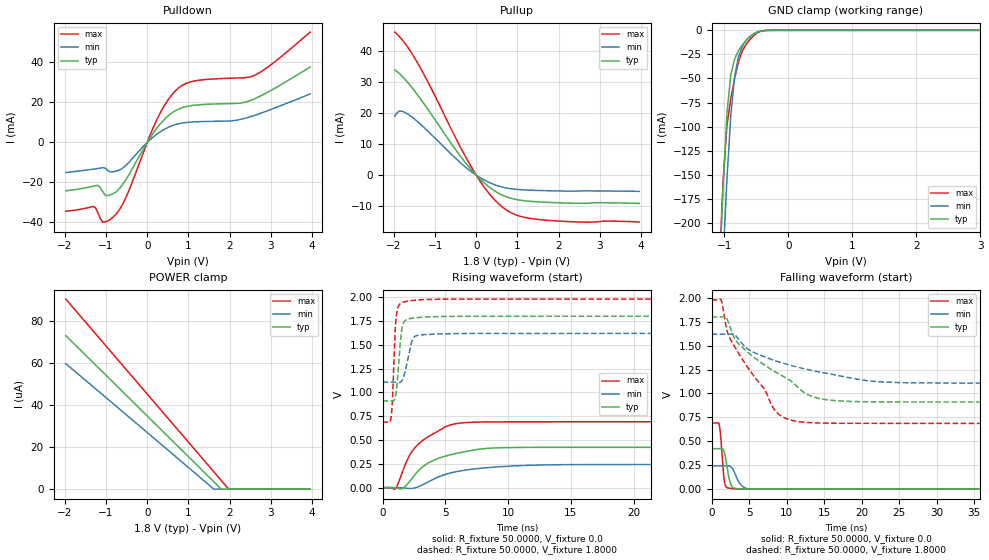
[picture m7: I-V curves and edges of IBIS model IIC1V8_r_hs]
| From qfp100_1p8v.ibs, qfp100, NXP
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[Model] IIC1V8_r_hs
|   Model IIC1V8_r_hs
| This model was characterised for following simulation conditions:
| External (pad) voltage:
|   - Typ: 1.8V,   - Min: 1.62V,   - Max: 1.98V
| Library cells for typ/min/max conditions are connected as defined below:
|  IO - External Pad
|  A - Core Input
|  EN - Output Buffer Enable
|  BOOST - vdde
|  EGP - vdd
|  EHS - vdd
|  ENZI - vdd
|  EPD - vdd
|  EPUN - gnd
|  ZI - NC
|  ZIF - NC
|  gnd - gnd
|  gnde - gnde
|  vdd - vdd
|  vdde - vdde
| All other pins connected to ground
Model_type I/O
Polarity   Non-Inverting
Enable   Active-Low
Vinl =   0.5400V
Vinh =   1.2600V
Vmeas =  0.9000V
Cref =   0.0F
Rref =   1.0000k
Vref =   0.0V
C_comp   3.6136pF   3.4665pF   3.7543pF
|C_comp_pullup   0.9376pF   0.9158pF   0.9440pF
|C_comp_pulldown   2.3253pF   2.4782pF   2.1796pF
[Model Spec]
| variable   typ   min   max
Vinh   0.5400V   0.4860V   0.5940V
Vinl   1.2600V   1.1340V   1.3860V
Vmeas   0.9000V   0.8100V   0.9900V
[Temperature Range]   25.0000   0.1250k   -40.0000
[Voltage Range]   1.8000V   1.6200V   1.9800V
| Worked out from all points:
|   slope of the pulldown table from 0 to 0.27 V, typ, clamps not added: 33.4 ohm
|   slope of the pullup table from 0 to 0.27 V, typ, clamps not added: 80.7 ohm
|   GND clamp passes 1 mA (typ) near -0.44 V on its own axis
|   rising waveform, R_fixture 50.0000, V_fixture 0.0: 20-80 % time 2.94ns typ, 3.7ns min, 2.37ns max; typ from 0 V to 0.423 V
|   rising waveform, R_fixture 50.0000, V_fixture 1.8000: 20-80 % time 334ps typ, 515ps min, 244ps max; typ from 0.91 V to 1.8 V
|   falling waveform, R_fixture 50.0000, V_fixture 0.0: 20-80 % time 581ps typ, 938ps min, 399ps max; typ from 0.423 V to 0 V
|   falling waveform, R_fixture 50.0000, V_fixture 1.8000: 20-80 % time 8.41ns typ, 11.2ns min, 5.74ns max; typ from 1.8 V to 0.91 V
[Pulldown]
|Voltage   I(typ)   I(min)   I(max)
-1.98V    -24.22mA   -15.04mA   -34.42mA
-1.32V    -21.94mA   -13.41mA   -32.06mA
-1.2V     -21.45mA   -13.05mA   -35.06mA
-1.08V    -24.63mA   -12.6mA    -39.9mA
-900mV    -26.23mA   -14.78mA   -38.53mA
-720mV    -24.07mA   -14.13mA   -34.99mA
-540mV    -19.33mA   -11.9mA    -28.53mA
300mV     8.856mA    5.096mA    14.12mA
720mV     16.26mA    9.117mA    26.48mA
1.14V     18.6mA     10.26mA    30.69mA
2.58V     21.55mA    13.34mA    33.32mA
3.96V     37.7mA     24.26mA    55.17mA
[Pullup]
|Voltage   I(typ)   I(min)   I(max)
-1.98V    33.82mA    18.95mA    45.98mA
-1.86V    32.54mA    20.66mA    44.41mA
-1.62V    29.1mA     19.25mA    40.23mA
-1.2V     21.63mA    14.45mA    30.58mA
-420mV    6.731mA    4.413mA    9.887mA
0V        -16.46nA   -7.885nA   -32.77nA
360mV     -4.265mA   -2.608mA   -6.666mA
660mV     -6.57mA    -3.917mA   -10.5mA
1.02V     -7.945mA   -4.606mA   -13.01mA
1.56V     -8.618mA   -4.934mA   -14.29mA
2.64V     -9.058mA   -5.064mA   -15.11mA
3.96V     -9.081mA   -5.209mA   -15.04mA
[GND_clamp]
|Voltage   I(typ)   I(min)   I(max)
-1.98V    -2.104A    -2.075A    -2.136A
-1.08V    -259.3mA   -333mA     -246.9mA
-1.02V    -161.8mA   -238.7mA   -157.1mA
-960mV    -86.75mA   -154.7mA   -99.47mA
-900mV    -45.96mA   -88.82mA   -71.06mA
-840mV    -29.91mA   -48mA      -50.26mA
-780mV    -21.16mA   -27.65mA   -32.99mA
-720mV    -15.17mA   -16.88mA   -21.27mA
-660mV    -10.57mA   -10.24mA   -14.57mA
-540mV    -3.796mA   -3.405mA   -5.301mA
-300mV    -21.69uA   -40.85uA   -23.15uA
3.96V     0A         0A         0A
[POWER_clamp]
|Voltage   I(typ)   I(min)   I(max)
-1.98V    73.06uA    59.72uA    90.42uA
1.62V     3.484uA    0A         8.225uA
1.8V      0A         0A         4.113uA
1.98V     0A         0A         0A
3.96V     0A         0A         0A
[Ramp]
| variable   typ   min   max
dV/dt_r  0.2537/2.9385n   0.1456/3.7026n   0.4146/2.3719n
dV/dt_f  0.5332/8.4056n   0.3066/11.2315n   0.7749/5.7392n
R_load = 50.0000
[Rising Waveform]
R_fixture= 50.0000
V_fixture= 0.0
V_fixture_min= 0.0
V_fixture_max= 0.0
|time   V(typ)   V(min)   V(max)
0s        583.8pV    50.78nV    39.11pV
1.054ns   -4.544mV   243uV      -9.405mV
1.612ns   -8.369mV   -2.334mV   175mV
2.288ns   86.03mV    -8.936mV   367.6mV
2.979ns   193.4mV    16.44mV    471mV
3.665ns   259.9mV    61.19mV    536.3mV
5.554ns   349.4mV    158.1mV    662.5mV
8.944ns   416.4mV    215.7mV    689.9mV
23.83ns   422.8mV    242.5mV    690.9mV
1us       422.9mV    242.6mV    691mV
[Rising Waveform]
R_fixture= 50.0000
V_fixture= 1.8000
V_fixture_min= 1.6200
V_fixture_max= 1.9800
|time   V(typ)   V(min)   V(max)
0s        910.3mV    1.108V     687.5mV
692.7ps   908.2mV    1.108V     745.4mV
790.9ps   905.2mV    1.109V     929.2mV
1.022ns   952.6mV    1.107V     1.685V
1.288ns   1.304V     1.102V     1.909V
1.517ns   1.647V     1.119V     1.94V
1.781ns   1.751V     1.21V      1.952V
2.544ns   1.781V     1.583V     1.967V
4.873ns   1.796V     1.614V     1.978V
1us       1.799V     1.619V     1.979V
[Falling Waveform]
R_fixture= 50.0000
V_fixture= 0.0
V_fixture_min= 0.0
V_fixture_max= 0.0
|time   V(typ)   V(min)   V(max)
0s        422.9mV    242.6mV    691mV
1.02ns    422.9mV    242.6mV    674.6mV
1.214ns   425.2mV    242.6mV    552.8mV
1.611ns   406.1mV    242.7mV    139.1mV
1.881ns   322.6mV    244.1mV    30.93mV
2.29ns    127.3mV    244.2mV    11.49mV
2.698ns   31.47mV    224mV      6.243mV
3.618ns   4.248mV    76.17mV    1.881mV
4.462ns   1.759mV    12.8mV     751.7uV
1us       17.18nV    79.91nV    9.929nV
[Falling Waveform]
R_fixture= 50.0000
V_fixture= 1.8000
V_fixture_min= 1.6200
V_fixture_max= 1.9800
|time   V(typ)   V(min)   V(max)
0s        1.799V     1.619V     1.979V
1.246ns   1.799V     1.619V     1.982V
1.896ns   1.801V     1.619V     1.715V
2.424ns   1.702V     1.621V     1.58V
3.741ns   1.509V     1.551V     1.402V
8.529ns   1.224V     1.342V     816mV
10.64ns   1.126V     1.292V     719.9mV
15.35ns   934.4mV    1.21V      689.9mV
35.17ns   910.7mV    1.109V     687.6mV
1us       910.3mV    1.108V     687.5mV
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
